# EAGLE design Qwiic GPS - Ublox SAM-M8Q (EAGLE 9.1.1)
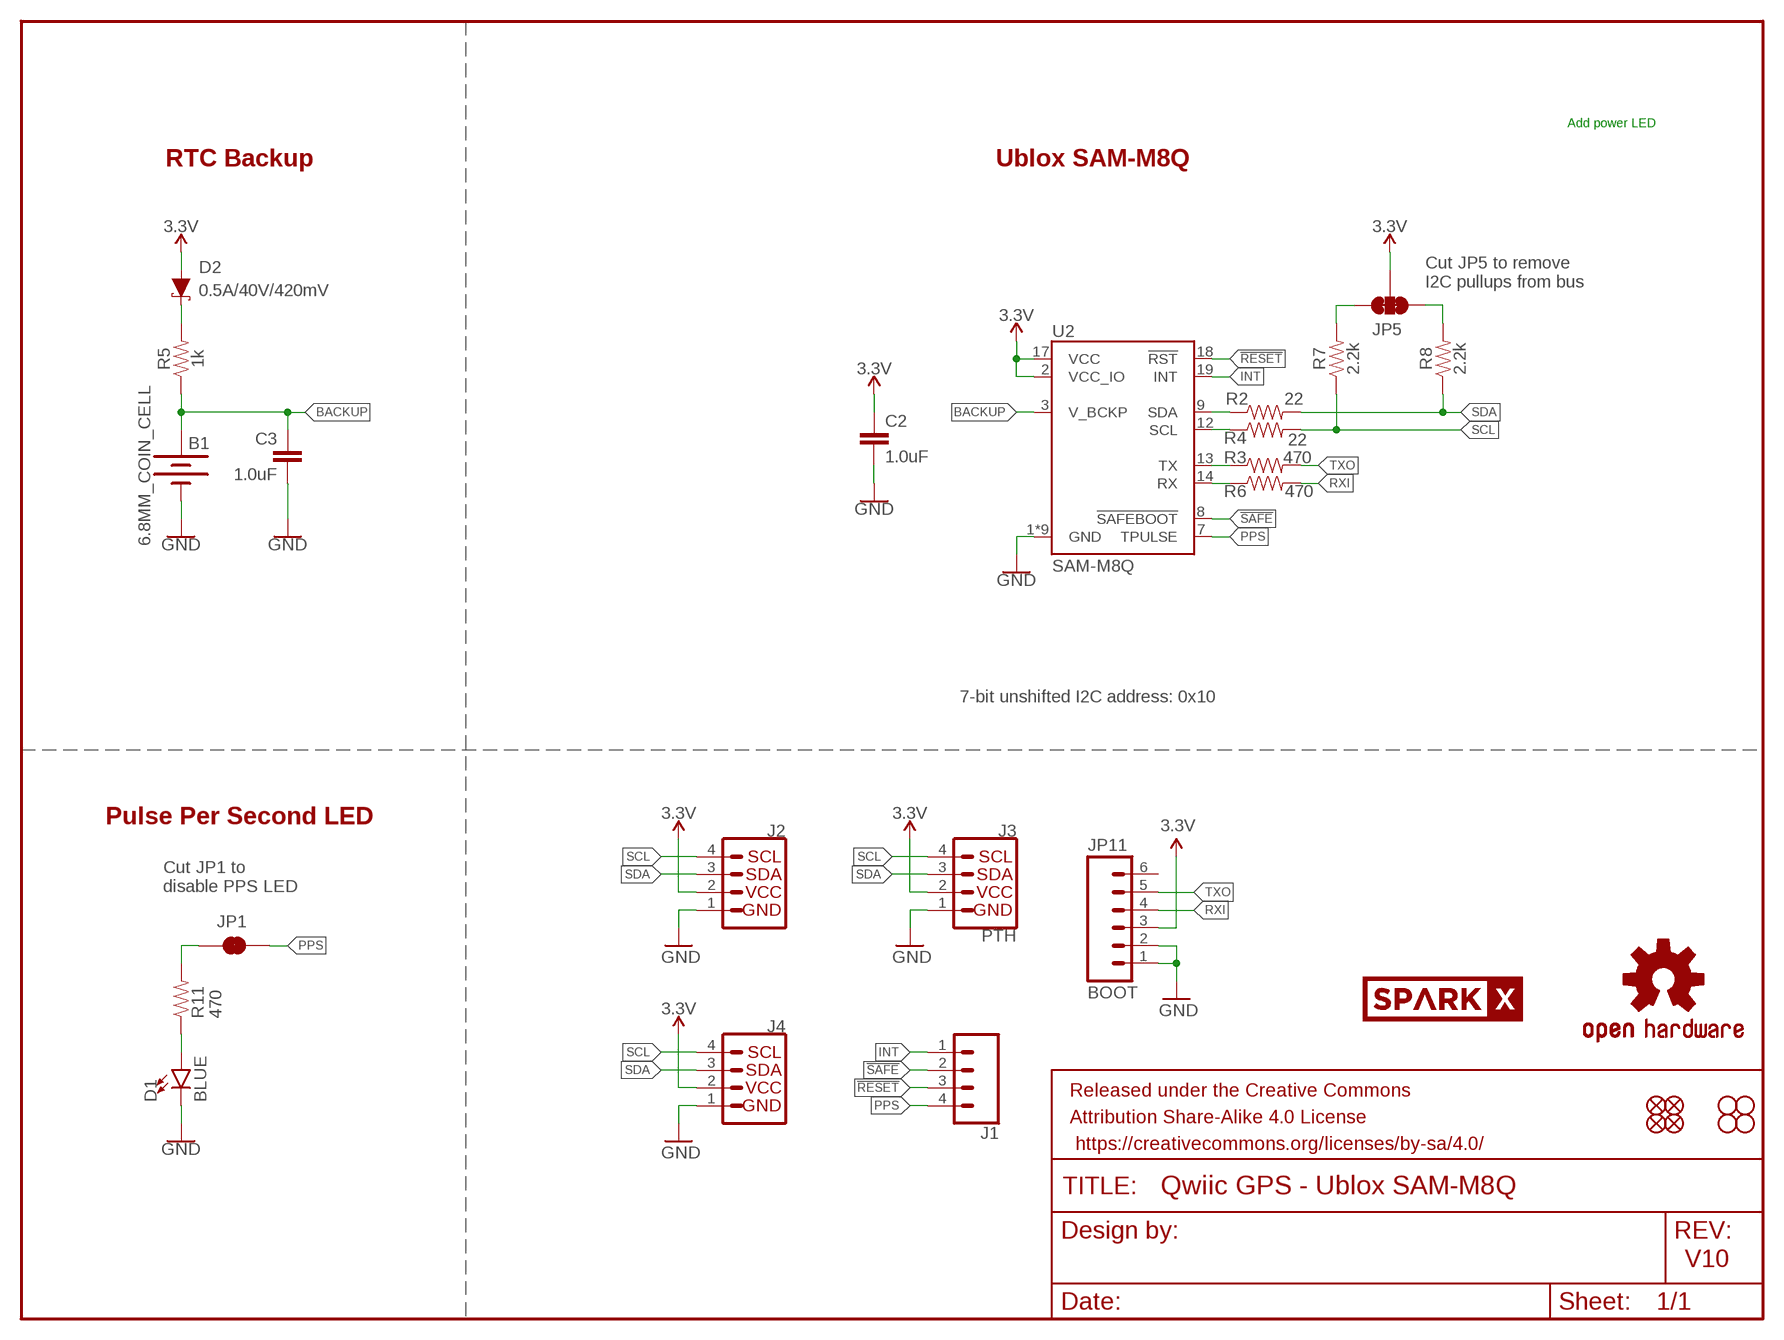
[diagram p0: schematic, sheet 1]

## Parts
B1  6.8MM_COIN_CELL  BATTERY-6.8MM_SMD  [BATTCON-6.8MM]
C2  1.0uF  1.0UF-0603-16V-10%  [0603]
C3  1.0uF  1.0UF-0603-16V-10%  [0603]
D1  BLUE  LED-BLUE0603  [LED-0603]
D2  0.5A/40V/420mV  DIODE-SCHOTTKY-PMEG4005EJ  [SOD-323]
FRAME1  FRAME-LETTER  [CREATIVE_COMMONS]
J1  CONN_041X04_NO_SILK  [1X04_NO_SILK]
J2  I2C_STANDARDQWIIC  [1X04_1MM_RA]
J3  PTH  I2C_STANDARD_NO_SILK  [1X04_NO_SILK]
J4  I2C_STANDARDQWIIC  [1X04_1MM_RA]
JP1  JUMPER-SMT_2_NC_TRACE_SILK  [SMT-JUMPER_2_NC_TRACE_SILK]
JP2  FIDUCIALUFIDUCIAL  [MICRO-FIDUCIAL]
JP3  STAND-OFF  [STAND-OFF]
JP4  STAND-OFF  [STAND-OFF]
JP5  JUMPER-SMT_3_2-NC_TRACE_SILK  [SMT-JUMPER_3_2-NC_TRACE_SILK]
JP6  FIDUCIALUFIDUCIAL  [MICRO-FIDUCIAL]
JP7  FIDUCIALUFIDUCIAL  [MICRO-FIDUCIAL]
JP8  FIDUCIALUFIDUCIAL  [MICRO-FIDUCIAL]
JP9  STAND-OFF  [STAND-OFF]
JP10  STAND-OFF  [STAND-OFF]
JP11  BOOT  M06NO_SILK_FEMALE_PTH  [1X06_NO_SILK]
LOGO1  OSHW-LOGOMINI  [OSHW-LOGO-MINI]
R2  22  22OHM-0603-1/10W-1%  [0603]
R3  470  470OHM-0603-1/10W-1%  [0603]
R4  22  22OHM-0603-1/10W-1%  [0603]
R5  1k  1KOHM-0603-1/10W-1%  [0603]
R6  470  470OHM-0603-1/10W-1%  [0603]
R7  2.2k  2.2KOHM-0603-1/10W-1%  [0603]
R8  2.2k  2.2KOHM-0603-1/10W-1%  [0603]
R11  470  470OHM-0603-1/10W-1%  [0603]
U2  SAM-M8Q  [SAM-M8Q]
U$31  SPARKX-LOGO4  [SPARKX-MEDIUM]

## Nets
3.3V: C2.1 D2.A J2.2 J3.2(VCC) J4.2 JP5.2 JP11.3 U2.2(VCC_IO) U2.17(VCC)
!RESET: J1.3 U2.18(!RST)
!SAFE: J1.2 U2.8(!SAFEBOOT)
BACKUP: B1.+ C3.1 R5.1 U2.3(V_BCKP)
GND: B1.- C2.2 C3.2 D1.C J2.1 J3.1(GND) J4.1 JP11.1 JP11.2 U2.1(GND) U2.4(GND) U2.5(GND) U2.6(GND) U2.10(GND) U2.11(GND) U2.15(GND) U2.16(GND) U2.20(GND)
INT: J1.1 U2.19(INT)
N$2: D1.A R11.1
N$4: JP1.1 R11.2
N$5: JP5.1 R8.2
N$6: D2.C R5.2
N$8: JP5.3 R7.2
PPS: J1.4 JP1.2 U2.7(TPULSE)
RXI: JP11.4 R6.2
RXLV: R6.1 U2.14(RX)
SCL: J2.4 J3.4(SCL) J4.4 R4.2 R7.1
SCL_LV: R4.1 U2.12(SCL)
SDA: J2.3 J3.3(SDA) J4.3 R2.2 R8.1
SDA_LV: R2.1 U2.9(SDA)
TXLV: R3.1 U2.13(TX)
TXO: JP11.5 R3.2
Unconnected: JP11.6

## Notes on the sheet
- Add power LED
- RTC Backup | Ublox SAM-M8Q
- Cut JP5 to remove 
  I2C pullups from bus
- 7-bit unshifted I2C address: 0x10
- Pulse Per Second LED
- Cut JP1 to 
  disable PPS LED
- V10

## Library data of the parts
B1 = SparkFun-Batteries:BATTERY: Battery - Single Cell; PROD_ID: BATT-13734
C2 C3 = SparkFun-Capacitors:1.0UF: 1µF ceramic capacitors; PROD_ID: CAP-00868
D1 = SparkFun-LED:LED-BLUE: Blue SMD LED; PROD_ID: DIO-08575
D2 = SparkFun-DiscreteSemi:DIODE-SCHOTTKY: Schottky diode; PROD_ID: DIO-10955
FRAME1 = SparkFun-Aesthetics:FRAME-LETTER: Schematic Frame - Letter
J1 = SparkFun-Connectors:CONN_04: Multi connection point. Often used as Generic Header-pin footprint for 0.1 inch spaced/style header connections On any of the 0.1 inch spaced packages, you can populate with these: Break Away Headers - Straight (PRT-00116) Break Away Male Headers - Right Angle (PRT-00553) Female Headers (PRT-00115)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; PROD_ID: CONN-09696
J2 J4 = SparkFun-Connectors:I2C_STANDARD: SparkFun I2C Standard Pinout Header SparkFun has standardized on a pinout for all I2C based sensor breakouts. This pinout allows I2C boards to be plugged directly into the headers on Arduino Uno compatible boards, and to be daisy chained easily. Example SparkFun Products: SparkFun Atmospheric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; PROD_ID: CONN-13694; VALUE: Qwiic Right Angle
J3 = SparkX:I2C_STANDARD: SparkFun I2C Standard Pinout Header SparkFun has standardized on a pinout for all I2C based sensor breakouts. This pinout allows I2C boards to be plugged directly into the headers on Arduino Uno compatible boards, and to be daisy chained easily. Example SparkFun Products: SparkFun Atmospheric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
JP1 = SparkFun-Jumpers:JUMPER-SMT_2_NC_TRACE: Normally closed trace jumper
JP2 JP6-JP8 = SparkFun:FIDUCIAL: Fiducial Alignment Points
JP3 JP4 JP9 JP10 = SparkFun:STAND-OFF: Stand Off
JP5 = SparkFun-Jumpers:JUMPER-SMT_3_2-NC_TRACE: Normally closed trace jumper (2 of 2 connections) This jumper has a trace between all three pads so they are normally closed (NC). Use a razor knife to open the connection(s). For best results follow the IPC guidelines for cutting traces: Cutout at least 0.063 mm (0.005 in). Remove all loose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
JP11 = SparkFun-Connectors:M06: Header 6 Standard 6-pin 0.1" header. Use with straight break away headers (SKU : PRT-00116), right angle break away headers (PRT-00553), swiss pins (PRT-00743), machine pins (PRT-00117), and female headers (PRT-00115). Molex polarized connector foot print use with SKU : PRT-08094 with associated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; PROD_ID: CONN-08437
LOGO1 = SparkFun-Aesthetics:OSHW-LOGO: Open-Source Hardware (OSHW) Logo
R2 R4 = SparkFun-Resistors:22OHM: 22Ω resistor; PROD_ID: RES-08698
R3 R6 R11 = SparkFun-Resistors:470OHM: 470Ω resistor; PROD_ID: RES-07869
R5 = SparkFun-Resistors:1KOHM: 1kΩ resistor; PROD_ID: RES-07856
R7 R8 = SparkFun-Resistors:2.2KOHM: 2.2kΩ resistor; PROD_ID: RES-08272
U2 = SAM-M8Q:SAM-M8Q
U$31 = SparkX:SPARKX-LOGO

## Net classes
1 vcc: width 0.152 mm

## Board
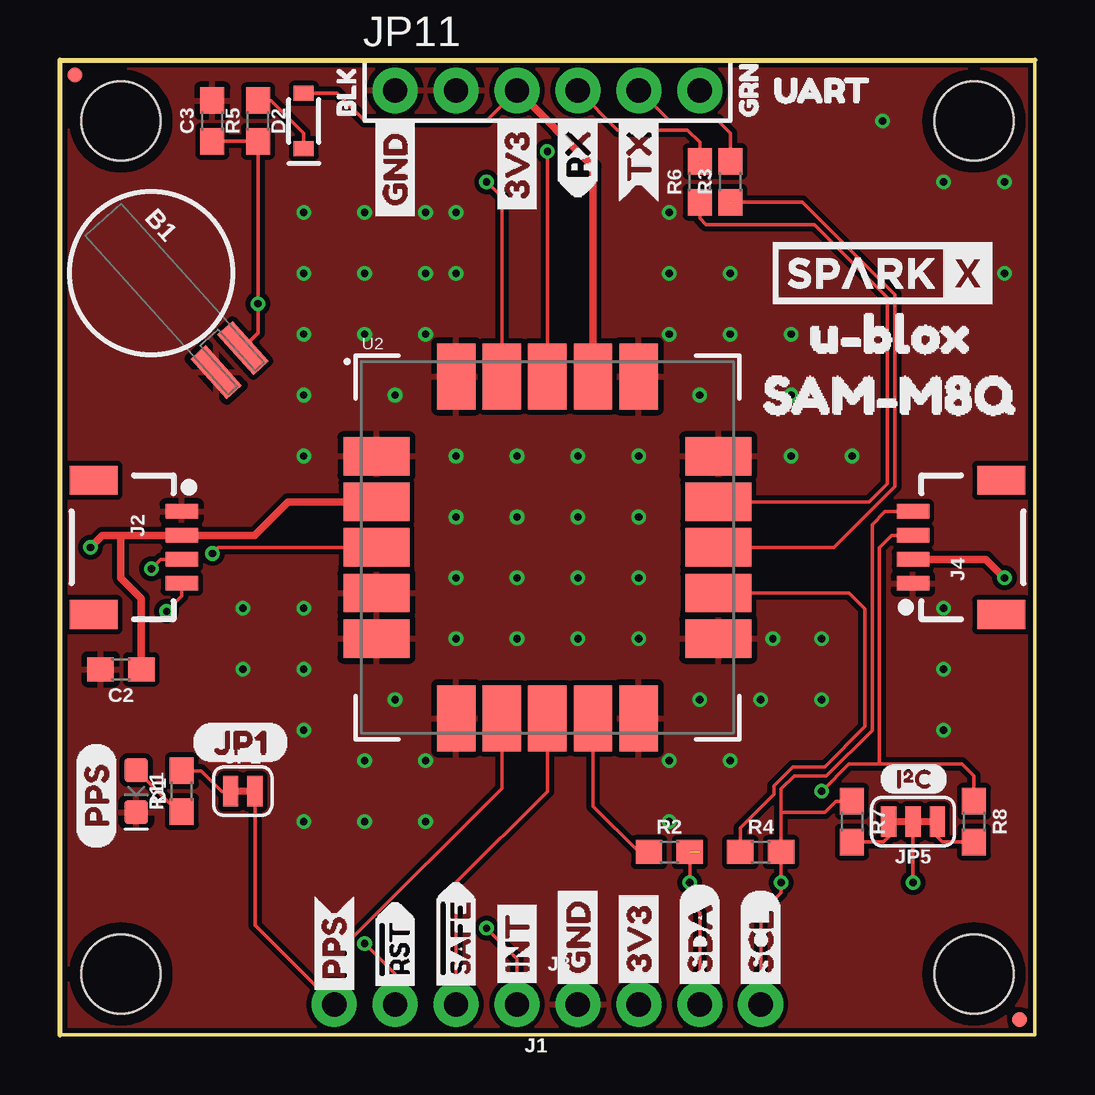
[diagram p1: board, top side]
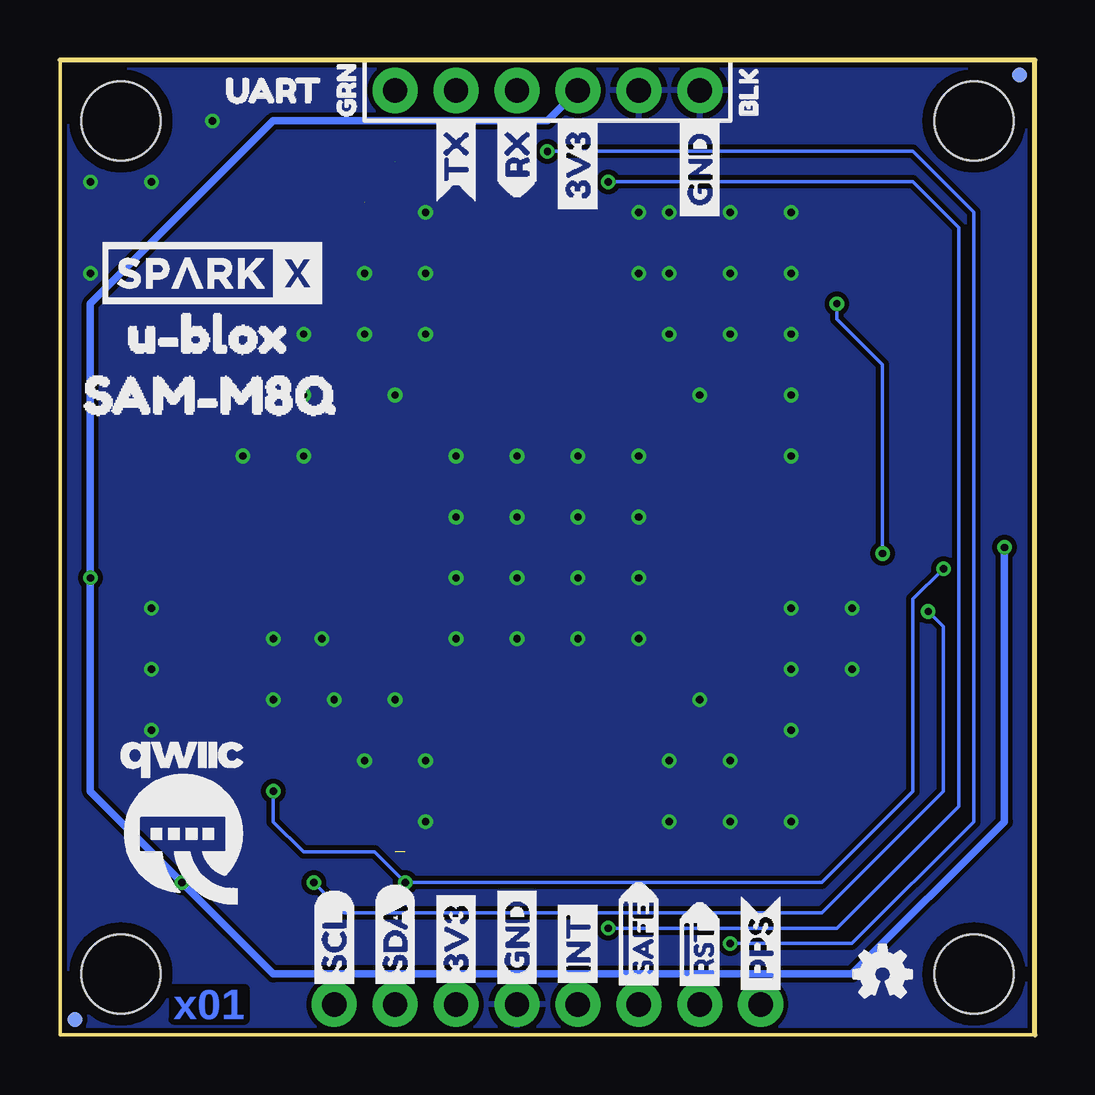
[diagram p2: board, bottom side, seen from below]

Size 40.64 x 40.64 mm. Coordinates in mm from the lower left corner, seen from the top.
Outline: 0,0 0,40.64 40.64,40.64 40.64,0 0,0
Copper layers (1*16): Top 0.035mm / dielectric 1.5mm / Bottom 0.035mm
Design rules "SparkFun-2-layer-PCBWay-LIMIT": minimum track width 6mil, minimum drill 0.3mm, track to track 6mil, track to pad 6mil, pad to pad 6mil, via to via 6mil, smd to smd 6mil, copper to edge 6mil, drill to drill 6mil, minimum pad ring 6mil, minimum via ring 6mil, stop-mask expansion 4mil, vias tented up to drill 25mil, thermal gap 10mil

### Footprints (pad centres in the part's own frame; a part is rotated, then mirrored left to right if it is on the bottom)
BATTCON-6.8MM = smd 2.25 x 0.85: + 4.87,0.75; - 4.87,-0.75
0603 = smd 1.1 x 1: 1 -0.85,0; 2 0.85,0
LED-0603 = smd 1 x 1: A -0.877,0; C 0.877,0
SOD-323 = smd 0.63 x 0.83: A 1.15,0; C -1.15,0
1X04_NO_SILK = drill 1.016 pad 1.88: 1 0,0; 2 2.54,0; 3 5.08,0; 4 7.62,0
1X04_1MM_RA = smd 0.6 x 1.35: 1 -1.5,0; 2 -0.5,0; 3 0.5,0; 4 1.5,0 | smd 1.2 x 2: NC1 2.8,-3.675; NC2 -2.8,-3.675
SMT-JUMPER_2_NC_TRACE_SILK = smd 0.635 x 1.27: 1 -0.508,0; 2 0.508,0
MICRO-FIDUCIAL = smd 0.635 x 0.635: 1 0,0
STAND-OFF = hole 3.302: 0,0
SMT-JUMPER_3_2-NC_TRACE_SILK = smd 0.635 x 1.27: 1 -1.016,0; 2 0,0; 3 1.016,0
1X06_NO_SILK = drill 1.016 pad 1.88: 1 0,0; 2 2.54,0; 3 5.08,0; 4 7.62,0; 5 10.16,0; 6 12.7,0
SAM-M8Q = smd 2.75 x 1.6: 1 -7.125,3.8; 2 -7.125,1.9; 3 -7.125,0; 4 -7.125,-1.9; 5 -7.125,-3.8; 11 7.125,-3.8; 12 7.125,-1.9; 13 7.125,0; 14 7.125,1.9; 15 7.125,3.8 | smd 1.6 x 2.75: 6 -3.8,-7.125; 7 -1.9,-7.125; 8 0,-7.125; 9 1.9,-7.125; 10 3.8,-7.125; 16 3.8,7.125; 17 1.9,7.125; 18 0,7.125; 19 -1.9,7.125; 20 -3.8,7.125

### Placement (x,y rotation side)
B1  3.81,31.75 312 top
C2  2.54,15.24 180 top
C3  6.35,38.1 90 top
D1  3.17,10.16 270 top
D2  10.16,38.1 90 top
FRAME1  not placed on the board
J1  19.05,1.27 180 top
J2  5.08,20.32 270 top
J3  21.59,1.27 0 top
J4  35.56,20.32 90 top
JP1  7.62,10.16 0 top
JP2  40.01,0.64 0 top
JP3  2.54,38.1 0 top
JP4  38.1,38.1 0 top
JP5  35.56,8.89 180 top
JP6  0.64,40.01 0 top
JP7  40.01,0.64 0 bottom
JP8  0.64,40.01 0 bottom
JP9  2.54,2.54 0 top
JP10  38.1,2.54 0 top
JP11  13.97,39.37 0 top
LOGO1  6.35,2.54 0 bottom
R2  25.4,7.62 0 top
R3  27.94,35.56 90 top
R4  29.21,7.62 0 top
R5  8.26,38.1 90 top
R6  26.67,35.56 90 top
R7  33.02,8.89 270 top
R8  38.1,8.89 270 top
R11  5.08,10.16 90 top
U2  20.32,20.32 0 top
U$1  [SDA-[)]  26.67,1.65 90 top
U$2  SPARKX-LOGO4  [SPARKX-MEDIUM]  34.29,31.75 0 bottom
U$3  [SCL-[)]  29.21,1.65 90 top
U$4  [SDA-[)]  26.67,1.65 90 bottom
U$5  [SCL-[)]  29.21,1.65 90 bottom
U$6  [3V3-04]  24.13,1.65 90 top
U$7  [3V3-04]  24.13,1.65 90 bottom
U$8  [GND-04]  21.59,1.65 90 top
U$9  [GND-04]  21.59,1.65 90 bottom
U$10  [I_SUPER2_C-()-03]  34.16,10.67 0 top
U$11  [UART0]  34.67,39.37 0 bottom
U$12  [BLK1]  11.94,37.59 90 top
U$13  [BLK1]  11.94,37.59 90 bottom
U$14  [GRN2]  28.7,37.59 90 top
U$15  [INT8]  19.05,1.65 90 top
U$16  [INT8]  19.05,1.65 90 bottom
U$17  [GRN2]  28.7,37.59 90 bottom
U$18  [JP10]  5.46,12.19 0 top
U$19  [RX6]  21.59,34.8 90 top
U$20  [RX6]  21.59,34.8 90 bottom
U$21  [SAM#M8Q4]  27.94,26.67 0 top
U$22  [U#BLOX3]  39.24,29.21 0 bottom
U$23  [TX7]  24.13,34.67 90 top
U$24  [TX7]  24.13,34.67 90 bottom
U$25  [SAM#M8Q4]  41.02,26.67 0 bottom
U$26  [U#BLOX3]  29.84,29.21 0 top
U$27  [3V3-04]  19.05,33.91 90 top
U$29  [PPS0]  1.52,7.75 90 top
U$30  [QWIIC-LOGO-MEDIUM]  35.56,8.89 0 bottom
U$31  34.29,31.75 0 top
U$32  [3V3-04]  19.05,33.91 90 bottom
U$33  [GND-04]  13.97,33.66 90 top
U$34  [GND-04]  13.97,33.66 90 bottom
U$35  [#RST3]  13.97,1.4 90 top
U$36  [#RST3]  13.97,1.4 90 bottom
U$39  [#SAFE1]  16.51,1.4 90 top
U$40  [#SAFE1]  16.51,1.4 90 bottom
U$43  [PPS5]  11.43,1.4 90 top
U$44  [PPS5]  11.43,1.4 90 bottom
U$45  [UART0]  28.83,39.37 0 top

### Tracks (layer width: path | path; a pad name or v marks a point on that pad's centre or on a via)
3.3V  (via drill 0.3)
  Top 0.152: D2.A 11.55,39.25 12.7,38.1 17.78,38.1 JP11.3 | J4.2 36.44,19.82 | JP5.2 v35.56,6.35
  Top 0.305: U2.2 9.52,22.22 8.12,20.82 J2.2 2.54,20.82 | v39.37,19.05 38.6,19.82 J4.2 | U2.17 22.22,36.2 JP11.3 | v1.27,20.32 1.77,20.82 2.54,20.82 | C2.1 3.39,18.2 2.54,19.05 2.54,20.82
  Bottom 0.305: JP11.3 20.32,38.1 31.75,38.1 39.37,30.48 v39.37,19.05 39.37,10.16 v35.56,6.35 31.75,2.54 24.13,2.54 | 24.13,2.54 7.62,2.54 1.27,8.89 v1.27,20.32 | J3.2 24.13,2.54
!RESET  (via drill 0.3)
  Top 0.152: v20.32,36.83 U2.18 | J1.3 13.97,2.54 v12.7,3.81
  Bottom 0.152: v12.7,3.81 7.62,3.81 2.54,8.89 2.54,34.29 5.08,36.83 v20.32,36.83
!SAFE
  Top 0.152: J1.2 16.51,6.35 20.32,10.16 U2.8
BACKUP  (via drill 0.3)
  Top 0.152: C3.1 R5.1 v8.26,30.48 8.26,29.26 B1.+ 8.2,29.21 | U2.3 6.6,20.32 v6.35,20.07
  Bottom 0.152: v6.35,20.07 6.35,27.94 8.26,29.84 v8.26,30.48
GND  (via drill 0.3)
  other vias: 16.51,24.13 19.05,24.13 21.59,24.13 24.13,24.13 16.51,19.05 19.05,19.05 21.59,19.05 24.13,19.05 16.51,21.59 19.05,21.59 21.59,21.59 24.13,21.59 10.16,17.78 10.16,15.24 10.16,12.7 12.7,11.43 13.97,13.97 26.67,13.97 26.67,26.67 13.97,26.67 10.16,24.13 10.16,26.67 10.16,29.21 12.7,29.21 27.94,29.21 30.48,29.21 30.48,26.67 30.48,24.13 27.94,11.43 25.4,11.43 15.24,11.43 15.24,29.21 25.4,29.21 34.29,38.1 36.83,35.56 39.37,35.56 39.37,31.75 36.83,12.7 36.83,15.24 16.51,16.51 19.05,16.51 21.59,16.51 24.13,16.51 16.51,31.75 12.7,31.75 10.16,31.75 25.4,31.75 27.94,31.75 25.4,34.29 29.21,13.97 31.75,13.97 31.75,16.51 29.72,16.51 36.83,17.78 33.02,24.13 16.51,34.29 12.7,34.29 10.16,34.29 15.24,31.75 15.24,34.29 15.24,8.89 12.7,8.89 10.16,8.89 7.62,17.78 7.62,15.24 25.4,8.89
  pour Bottom (isolate 0.305): 
  pour Top (isolate 0.305, rank 2): 
  pour Top (isolate 0.203): 0,40.64 40.64,40.64 40.64,0 0,0
  pour Bottom (isolate 0.203): 0,40.64 40.64,40.64 40.64,0 0,0
INT  (via drill 0.3)
  Top 0.152: v17.78,35.56 18.42,34.92 U2.19 | J1.1 19.05,3.17 v17.78,4.45
  Bottom 0.152: v17.78,4.45 8.26,4.45 3.17,9.53 3.17,33.66 5.08,35.56 v17.78,35.56
N$2
  Top 0.152: R11.1 4.9,9.31 D1.A
N$4
  Top 0.152: JP1.1 6.73,10.16 5.88,11.01 R11.2
N$5
  Top 0.152: R8.2 36.79,8.04 36.58,8.26 JP5.1
N$6
  Top 0.152: R5.2 8.8,38.95 10.16,37.59 D2.C
N$8
  Top 0.152: R7.2 34.33,8.04 34.54,8.26 JP5.3
PPS
  Top 0.152: JP1.2 8.13,4.57 J1.4 12.17,2.01 12.17,4.03 18.42,10.28 U2.7
RXI  (1 unrouted)
  Top 0.152: JP11.4 23.24,37.72 26.16,37.72 26.67,37.21 R6.2
RXLV
  Top 0.152: U2.14 33.73,22.22 34.49,22.99 34.49,30.73 31.45,33.78 26.92,33.78 26.67,34.04 R6.1
SCL  (via drill 0.3)
  Top 0.152: J3.4 29.21,5.08 30.06,5.93 R4.2 | v30.06,6.35 R4.2 | J2.4 5.08,18.29 v4.45,17.65 | J4.4 34.39,21.82 33.86,21.29 33.86,12.7 31.95,10.79 30.61,10.79 30.06,10.25 30.06,9.27 | R4.2 30.06,9.27 | R7.1 32.35,9.74 31.88,9.27 30.06,9.27
  Bottom 0.152: v4.45,17.65 3.81,17.02 3.81,10.16 8.89,5.08 28.79,5.08 v30.06,6.35
SCL_LV
  Top 0.152: R4.1 28.36,8.64 29.75,10.03 29.75,10.37 30.56,11.18 31.88,11.18 33.55,12.85 33.55,17.75 32.89,18.42 U2.12
SDA  (via drill 0.3)  (1 unrouted)
  Top 0.152: J3.3 26.67,5.08 26.25,5.5 v26.25,6.35 R2.2 | 26.67,7.62 26.25,8.04 | R8.1 38.1,10.79 37.59,11.3 34.16,11.3 | v3.81,19.43 4.2,19.82 J2.3 | J4.3 34.66,20.82 34.16,20.32 34.16,11.3 | v31.75,10.16 32.89,11.3 34.16,11.3
  Bottom 0.152: v3.81,19.43 5.08,18.16 5.08,10.16 8.89,6.35 v26.25,6.35 27.52,7.62 30.48,7.62 31.75,8.89 v31.75,10.16
SDA_LV
  Top 0.152: U2.9 22.22,9.53 24.13,7.62 R2.1
TXLV  (1 unrouted)
  Top 0.152: R3.1 30.95,34.71 32,33.66 34.8,30.86 34.8,22.86 32.26,20.32 U2.13
TXO
  Top 0.152: JP11.5 25.4,38.1 27.43,38.1 27.94,37.59 R3.2

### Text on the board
Bottom: x01
Measures: Measurements in inches

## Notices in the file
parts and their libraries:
SparkFun-Resistors: Licensing: Creative Commons ShareAlike 4.0 International - https://creativecommons.org/licenses/by-sa/4.0
SparkFun-Aesthetics: Released under the Creative Commons Attribution Share-Alike 4.0 License
SparkFun-Aesthetics: https://creativecommons.org/licenses/by-sa/4.0
